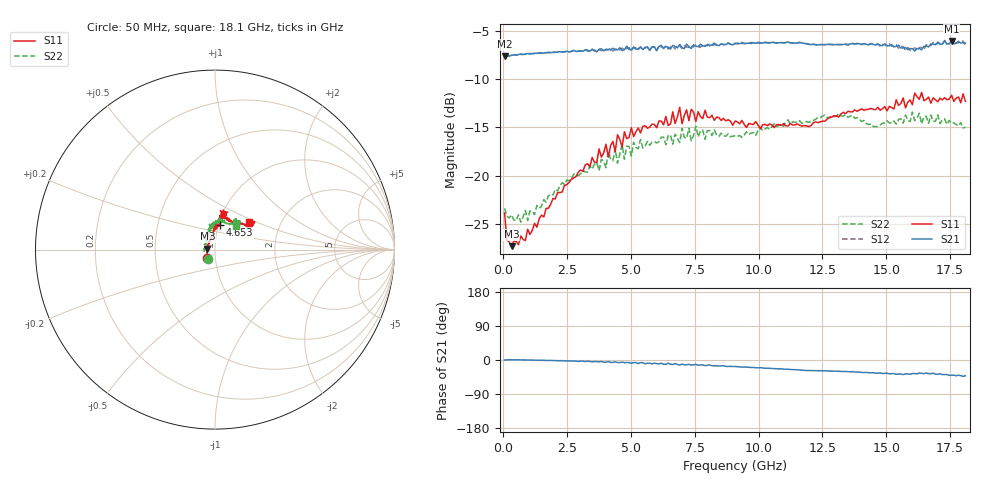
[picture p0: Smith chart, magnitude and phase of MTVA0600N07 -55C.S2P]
! Network Analyzer HP8720D.06.14 Serial No. US36140669
!  6 Jul 2005  09:17:12
! Frequency  S11  S21  S12  S22
# HZ  S  DB R 50
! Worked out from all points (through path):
!   201 points, 50 MHz to 18.1 GHz, reference 50 ohm
!   highest |S21| = -6.07 dB at 17.56 GHz (marker M1); lowest = -7.6 dB at 50 MHz (marker M2)
!   group delay of S21, straight-line fit = 7.03 ps
!   lowest |S11| = -27.3 dB at 320.8 MHz (marker M3), VSWR 1.09, Z = 45.9 + j0.471 ohm
!   |S11| at or under -10 dB: start of sweep to end of sweep
!   |S22| runs from -24.8 to -13.4 dB; largest |S21 - S12| = 0.023
!   S11 on the Smith chart (normalised r, x): 50 MHz: 0.91, -0.09; 4.653 GHz: 1.01, +0.29; 18.1 GHz: 1.38, +0.45
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5e7  -23.88 -132.6  -7.64 0.0  -7.64 0.0  -23.40 -126.4
1.4025e8  -26.71 -163.3  -7.62 0.3  -7.62 0.4  -24.20 -165.7
3.2075e8  -27.31 173.2  -7.55 0.6  -7.56 0.5  -24.08 175.2
9.525e8  -25.56 135.5  -7.37 0.2  -7.42 0.2  -24.65 147.8
3.1185e9  -19.56 93.4  -7.13 -3.1  -7.16 -3.6  -19.50 110.9
4.021e9  -16.75 87.3  -6.91 -5.7  -7.03 -4.5  -19.20 101.8
4.382e9  -17.55 83.8  -6.97 -4.8  -6.92 -6.5  -17.23 101.0
4.47225e9  -15.78 79.0  -6.99 -6.7  -6.87 -5.2  -18.72 104.3
4.65275e9  -17.05 78.9  -7.06 -5.5  -6.81 -6.8  -16.81 102.6
4.743e9  -15.47 81.8  -6.99 -7.1  -6.96 -5.9  -18.31 98.5
5.104e9  -15.96 83.5  -6.68 -6.8  -6.76 -8.0  -16.55 93.6
6.09675e9  -14.35 77.3  -6.64 -10.2  -6.57 -9.9  -16.49 89.2
6.7285e9  -14.61 81.5  -6.63 -9.3  -6.89 -10.5  -15.71 82.3
6.909e9  -12.94 78.1  -6.42 -13.1  -6.60 -11.3  -16.59 80.3
6.99925e9  -14.63 78.0  -6.74 -11.0  -6.84 -13.1  -15.12 81.3
7.36025e9  -13.13 71.4  -6.85 -13.4  -6.58 -12.1  -16.40 84.6
7.54075e9  -14.40 72.4  -6.59 -11.5  -6.45 -14.2  -14.89 83.0
9.075e9  -14.36 72.2  -6.33 -17.3  -6.31 -17.4  -15.88 68.1
1.21435e10  -14.53 50.9  -6.42 -27.8  -6.38 -27.8  -14.30 56.8
1.512175e10  -12.84 31.9  -6.56 -36.5  -6.37 -36.1  -14.54 52.6
1.75585e10  -11.69 39.1  -6.07 -40.1  -6.10 -39.9  -14.60 52.8
1.81e10  -12.31 38.8  -6.28 -41.6  -6.49 -42.1  -15.00 48.3
